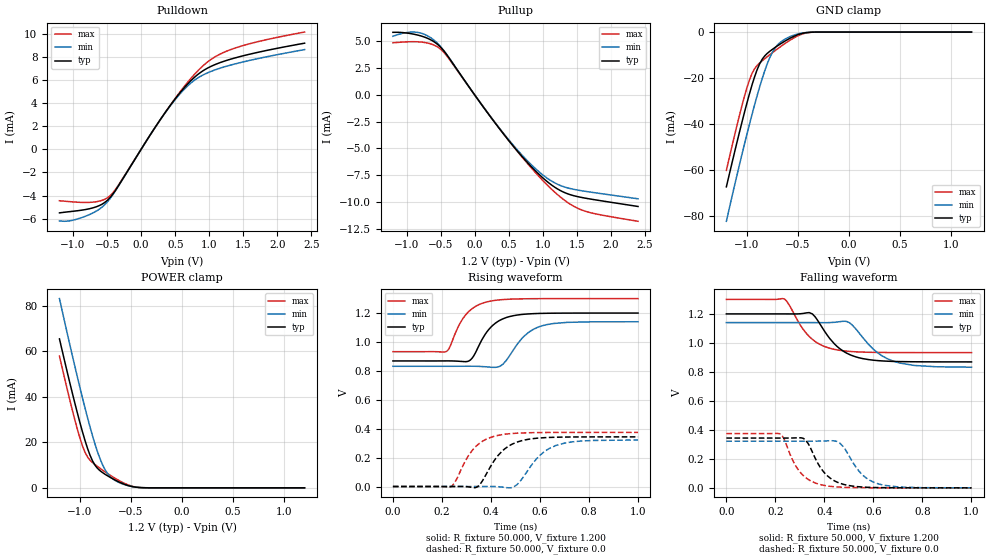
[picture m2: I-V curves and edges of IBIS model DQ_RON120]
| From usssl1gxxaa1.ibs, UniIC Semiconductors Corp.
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|   Model DQ_RON120
[Model] DQ_RON120
Model_type I/O
Vinl =  0.500V
Vinh =  0.700V
Vmeas =  0.600V
Rref =  50.000
Vref =  0.600V
C_comp   1.373pF   1.353pF   1.403pF
[Model Spec]
Vinh   0.700V   0.670V   0.750V
Vinl   0.500V   0.470V   0.550V
Vmeas   0.600V   0.570V   0.650V
Vref   0.600V   0.570V   0.650V
Rref   50.000   NA   NA
[Temperature Range]   25.000   0.125k   -40.000
[Voltage Range]   1.200V   1.140V   1.300V
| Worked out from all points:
|   slope of the pulldown table from 0 to 0.18 V, typ, clamps not added: 108 ohm
|   slope of the pullup table from 0 to 0.18 V, typ, clamps not added: 113 ohm
|   GND clamp passes 1 mA (typ) near -0.49 V on its own axis
|   POWER clamp passes 1 mA (typ) near -0.53 V on its own axis
|   rising waveform, R_fixture 50.000, V_fixture 1.200: 20-80 % time 81.5ps typ, 93.1ps min, 78.4ps max; typ from 0.869 V to 1.2 V
|   rising waveform, R_fixture 50.000, V_fixture 0.0: 20-80 % time 92.6ps typ, 101ps min, 87.1ps max; typ from 0 V to 0.343 V
|   falling waveform, R_fixture 50.000, V_fixture 1.200: 20-80 % time 104ps typ, 117ps min, 97.4ps max; typ from 1.2 V to 0.869 V
|   falling waveform, R_fixture 50.000, V_fixture 0.0: 20-80 % time 79.1ps typ, 86.1ps min, 75.9ps max; typ from 0.343 V to 0 V
[Pulldown]
|Voltage   I(typ)   I(min)   I(max)
-1.2V     -5.501mA   -6.195mA   -4.453mA
-1.015V   -5.372mA   -6.152mA   -4.547mA
-756mV    -5.139mA   -5.641mA   -4.594mA
-571mV    -4.739mA   -4.988mA   -4.412mA
-460mV    -4.203mA   -4.294mA   -4.038mA
-349mV    -3.3mA     -3.329mA   -3.237mA
354mV     3.185mA    3.161mA    3.186mA
613mV     5.183mA    5.063mA    5.279mA
798mV     6.299mA    6.032mA    6.57mA
1.02V     7.148mA    6.718mA    7.743mA
1.316V    7.79mA     7.28mA     8.618mA
2.4V      9.17mA     8.616mA    10.13mA
[Pullup]
|Voltage   I(typ)   I(min)   I(max)
-1.2V     5.842mA    5.474mA    4.866mA
-1.004V   5.781mA    5.816mA    4.949mA
-819mV    5.558mA    5.816mA    4.949mA
-634mV    5.104mA    5.29mA     4.739mA
-486mV    4.358mA    4.405mA    4.193mA
106mV     -945.3uA   -938.5uA   -932.8uA
513mV     -4.365mA   -4.294mA   -4.365mA
846mV     -6.8mA     -6.612mA   -6.924mA
1.142V    -8.479mA   -8.103mA   -8.89mA
1.364V    -9.242mA   -8.693mA   -10.05mA
1.586V    -9.607mA   -8.976mA   -10.79mA
2.4V      -10.43mA   -9.715mA   -11.81mA
[GND_clamp]
|Voltage   I(typ)   I(min)   I(max)
-1.2V     -67.26mA   -82.22mA   -60.1mA
-1.05V    -39.62mA   -53.62mA   -32.4mA
-1V       -31.05mA   -44.64mA   -24.37mA
-950mV    -23.16mA   -36.01mA   -18.1mA
-925mV    -19.62mA   -31.85mA   -16.02mA
-875mV    -13.89mA   -23.97mA   -13.48mA
-800mV    -9.288mA   -13.81mA   -10.72mA
-750mV    -7.535mA   -8.829mA   -8.993mA
-675mV    -5.274mA   -4.578mA   -6.506mA
-525mV    -1.587mA   -1.138mA   -2.208mA
-375mV    -90.13uA   -87.27uA   -132.9uA
1.2V      0A         0A         0A
[POWER_clamp]
|Voltage   I(typ)   I(min)   I(max)
-1.2V     65.51mA    83.21mA    57.91mA
-1.05V    37.38mA    53.57mA    29.99mA
-1V       28.74mA    44.18mA    21.95mA
-950mV    20.85mA    35.16mA    15.65mA
-925mV    17.34mA    30.84mA    13.56mA
-875mV    11.74mA    22.7mA     11.06mA
-800mV    7.436mA    12.47mA    8.502mA
-750mV    5.864mA    7.69mA     6.933mA
-675mV    3.901mA    3.837mA    4.735mA
-525mV    971.5uA    903.1uA    1.25mA
-400mV    85.95uA    125.9uA    91.19uA
1.2V      0A         0A         0A
[Ramp]
| variable   typ   min   max
dV/dt_r   0.206/92.488p   0.193/0.101n   0.225/87.374p
dV/dt_f   0.199/0.105n   0.185/0.117n   0.220/97.570p
R_load = 50.000
[Rising Waveform]
R_fixture= 50.000
V_fixture= 1.200
V_fixture_min= 1.140
V_fixture_max= 1.300
|time   V(typ)   V(min)   V(max)
0s        868.7mV    831.8mV    932.8mV
218ps     869mV      831.8mV    934.3mV
229ps     869mV      831.8mV    954.7mV
278ps     865.5mV    832mV      1.142V
316ps     875.2mV    832.2mV    1.221V
390ps     1.084V     826.8mV    1.28V
449ps     1.16V      846.6mV    1.293V
534ps     1.192V     1.038V     1.299V
604ps     1.198V     1.11V      1.3V
1ns       1.2V       1.14V      1.3V
[Rising Waveform]
R_fixture= 50.000
V_fixture= 0.0
V_fixture_min= 0.0
V_fixture_max= 0.0
|time   V(typ)   V(min)   V(max)
0s        62.39nV    1.09uV     36.07nV
238ps     82.91uV    -4.09uV    103.7uV
303ps     -1.391mV   -15.94uV   199.2mV
342ps     -4.396mV   146.7uV    283.1mV
422ps     199.8mV    -480.1uV   351.3mV
505ps     306.5mV    11.15mV    368.8mV
598ps     335.7mV    212.8mV    373.3mV
666ps     341mV      284.5mV    374mV
770ps     343mV      315mV      374.3mV
1ns       343.4mV    321.8mV    374.4mV
[Falling Waveform]
R_fixture= 50.000
V_fixture= 1.200
V_fixture_min= 1.140
V_fixture_max= 1.300
|time   V(typ)   V(min)   V(max)
0s        1.2V       1.14V      1.3V
234ps     1.2V       1.14V      1.304V
314ps     1.203V     1.14V      1.092V
351ps     1.2V       1.14V      1.024V
441ps     992.8mV    1.142V     955mV
501ps     920.8mV    1.14V      941.5mV
600ps     880.6mV    955.9mV    934.6mV
677ps     872.4mV    876.3mV    933.4mV
767ps     869.6mV    844.2mV    933mV
1ns       868.7mV    832.2mV    932.9mV
[Falling Waveform]
R_fixture= 50.000
V_fixture= 0.0
V_fixture_min= 0.0
V_fixture_max= 0.0
|time   V(typ)   V(min)   V(max)
0s        343.5mV    321.9mV    374.4mV
221ps     343.3mV    321.9mV    369.9mV
237ps     343.2mV    321.9mV    331.1mV
282ps     344.5mV    321.8mV    153.9mV
321ps     333.3mV    321.6mV    73.84mV
388ps     129.3mV    322.8mV    20.63mV
461ps     32.98mV    311.2mV    5.176mV
548ps     6.394mV    101.3mV    986.3uV
624ps     1.508mV    25.29mV    230.4uV
1ns       1.245uV    23.77uV    209.4nV
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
